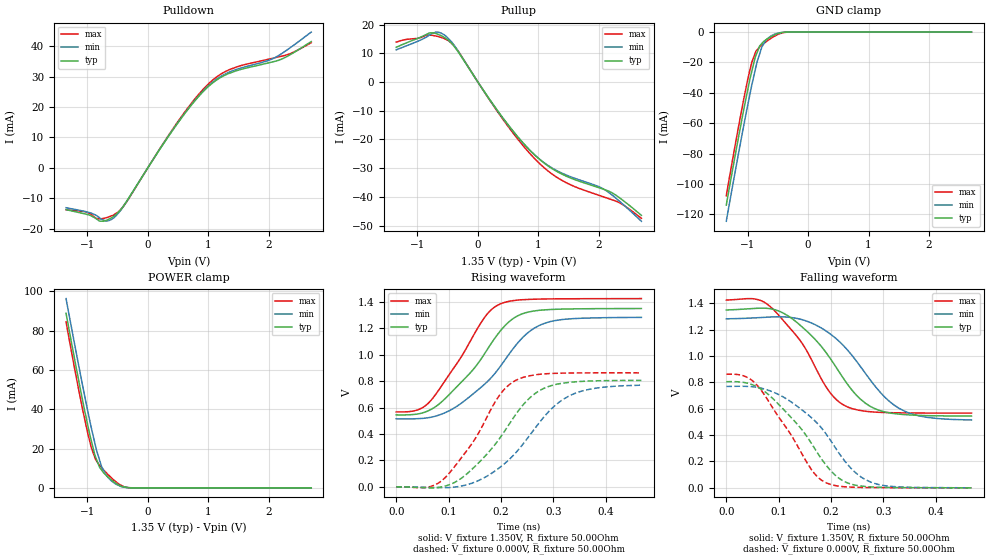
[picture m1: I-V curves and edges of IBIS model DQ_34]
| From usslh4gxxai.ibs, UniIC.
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| MODEL DQ_34 (34 Ohm Data I/O with no ODT, 800-2133Mbps)
[Model]   DQ_34
Model_type   I/O
Vinl = 545.000mV
Vinh = 805.000mV
Vmeas = 675.000mV
Vref = 675.000mV
Cref = 0.0pF
Rref = 25.000Ohm
|   typ   min   max
|C_comp   0.950pF   0.900pF   1.000pF
C_comp_pullup   0.4750pF   0.4500pF   0.5000pF
C_comp_pulldown   0.4750pF   0.4500pF   0.5000pF
[Model Spec]
| Input threshold voltage corners
Vinl   0.5450V   0.5115V   0.5825V
Vinh   0.8050V   0.7715V   0.8425V
| Measurement voltage corners
Vmeas   0.6750V   0.6415V   0.7125V
| Timing spec test load voltage corners
Vref   0.6750V   0.6415V   0.7125V
| Dynamic Overshoot Parameters from DDR3L Specification
|D_overshoot_ampl_h   0.40   NA   NA
|D_overshoot_ampl_l   0.40   NA   NA
|D_overshoot_area_h   0.11n   NA   NA
|D_overshoot_area_l   0.11n   NA   NA
[Receiver Thresholds]
Vth   =  0.675V
Vth_min  =  0.6615V
Vth_max  =  0.6885V
Vinh_ac  =  0.130V
Vinh_dc  =  0.090V
Vinl_ac  = -0.130V
Vinl_dc  = -0.090V
Tslew_ac =  5.000ns |Not specified, so set to high value
Threshold_sensitivity = 0.50
Reference_supply Pullup_ref
[Voltage Range]   1.3500V   1.2830V   1.4250V
[Pullup Reference]   1.3500V   1.2830V   1.4250V
[Temperature Range]   45.0   95.0   -40.0
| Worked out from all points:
|   slope of the pulldown table from 0 to 0.203 V, typ, clamps not added: 32.4 ohm
|   slope of the pullup table from 0 to 0.203 V, typ, clamps not added: 32.1 ohm
|   GND clamp passes 1 mA (typ) near -0.50 V on its own axis
|   POWER clamp passes 1 mA (typ) near -0.45 V on its own axis
|   falling waveform, V_fixture 1.350V, R_fixture 50.00Ohm: 20-80 % time 94.1ps typ, 97.5ps min, 82.7ps max; typ from 1.35 V to 0.545 V
|   rising waveform, V_fixture 1.350V, R_fixture 50.00Ohm: 20-80 % time 97.8ps typ, 105ps min, 81.4ps max; typ from 0.545 V to 1.35 V
|   rising waveform, V_fixture 0.000V, R_fixture 50.00Ohm: 20-80 % time 95.5ps typ, 103ps min, 81.4ps max; typ from 0 V to 0.806 V
|   falling waveform, V_fixture 0.000V, R_fixture 50.00Ohm: 20-80 % time 95.4ps typ, 100ps min, 81.6ps max; typ from 0.806 V to 0 V
[Pulldown]
|   Voltage   I(typ)   I(min)   I(max)
-1.35V    -13.75mA   -13.12mA   -13.81mA
-1V       -15.34mA   -14.53mA   -14.6mA
-800mV    -17.5mA    -16.38mA   -16.81mA
-690mV    -17.29mA   -17.5mA    -16.42mA
-565mV    -15.95mA   -16.5mA    -15.5mA
-395mV    -12.31mA   -12.44mA   -12.52mA
560mV     16.52mA    16.6mA     16.96mA
1.055V    27.67mA    27.92mA    28.56mA
1.465V    31.94mA    32.36mA    33.16mA
2.105V    35.05mA    36.27mA    36.22mA
2.34V     37.07mA    39.31mA    37.44mA
2.7V      41.52mA    44.64mA    41.15mA
[GND Clamp]
|   Voltage   I(typ)   I(min)   I(max)
-1.35V    -113.9mA   -124.5mA   -107.8mA
-1.205V   -81.48mA   -92.16mA   -74.7mA
-1.07V    -52.65mA   -63.14mA   -45.67mA
-1V       -38.7mA    -48.81mA   -31.8mA
-930mV    -25.95mA   -35.03mA   -20mA
-875mV    -16.88mA   -25.36mA   -14.11mA
-800mV    -9.222mA   -14.41mA   -9.781mA
-765mV    -7.604mA   -9.974mA   -8.618mA
-650mV    -3.918mA   -3.687mA   -5.173mA
-485mV    -837.4uA   -633.1uA   -1.288mA
-315mV    -19.67uA   -18.79uA   -29.52uA
2.7V      0A         0A         0A
[Pullup]
|   Voltage   I(typ)   I(min)   I(max)
-1.35V    12.15mA    11.27mA    13.95mA
-800mV    17.18mA    16.42mA    16.44mA
-690mV    16.9mA     17.47mA    16.07mA
-565mV    15.71mA    16.61mA    15.28mA
-320mV    10.4mA     10.59mA    10.63mA
470mV     -14.09mA   -14.2mA    -14.64mA
775mV     -21.88mA   -21.96mA   -22.88mA
1.055V    -27.57mA   -27.49mA   -29.11mA
1.465V    -32.85mA   -32.46mA   -35.14mA
2.105V    -37.57mA   -37.65mA   -40.24mA
2.34V     -40.35mA   -41.55mA   -42.07mA
2.7V      -46.46mA   -48.52mA   -47.48mA
[POWER Clamp]
|   Voltage   I(typ)   I(min)   I(max)
-1.35V    88.89mA    96.37mA    84.56mA
-1.205V   64.87mA    72.5mA     60.12mA
-1.07V    43.46mA    51mA       38.94mA
-930mV    23.58mA    30.09mA    20.17mA
-875mV    16.77mA    22.82mA    15.5mA
-800mV    10.68mA    14.43mA    11.57mA
-765mV    9.147mA    10.97mA    10.32mA
-690mV    6.433mA    6.617mA    7.805mA
-565mV    3.162mA    2.653mA    4.047mA
-395mV    485.8uA    358.5uA    553.6uA
-310mV    60.31uA    60.42uA    68.78uA
2.7V      0A         0A         0A
[Ramp]
R_load = 50.00Ohm
|   typ   min   max
dV/dt_r   483.363mV/95.498ps  461.741mV/103.129ps 517.629mV/81.416ps
dV/dt_f   483.183mV/94.118ps  460.840mV/97.492ps  514.663mV/82.746ps
[Falling Waveform]
V_fixture = 1.350V
V_fixture_min = 1.283V
V_fixture_max = 1.425V
R_fixture = 50.00Ohm
|   Time   V(typ)   V(min)   V(max)
0s        1.35V      1.283V     1.425V
54ps      1.362V     1.29V      1.434V
84ps      1.359V     1.296V     1.375V
162ps     1.157V     1.252V     977.6mV
198ps     984.4mV    1.169V     722.9mV
230ps     793.7mV    1.052V     616.4mV
274ps     620mV      823mV      577.8mV
328ps     560.3mV    607.7mV    569.4mV
382ps     548.1mV    535.9mV    567.6mV
468ps     544.7mV    514.9mV    567.2mV
[Rising Waveform]
V_fixture = 1.350V
V_fixture_min = 1.283V
V_fixture_max = 1.425V
R_fixture = 50.00Ohm
|   Time   V(typ)   V(min)   V(max)
0s        544.7mV    514.9mV    567.2mV
38ps      549.8mV    515.5mV    578.9mV
64ps      581mV      525.1mV    644.1mV
122ps     783.2mV    626.6mV    970.4mV
168ps     1.004V     774.3mV    1.279V
198ps     1.176V     907.7mV    1.383V
232ps     1.295V     1.089V     1.414V
280ps     1.339V     1.233V     1.422V
336ps     1.347V     1.273V     1.424V
468ps     1.35V      1.283V     1.425V
[Rising Waveform]
V_fixture = 0.000V
V_fixture_min = 0.000V
V_fixture_max = 0.000V
R_fixture = 50.00Ohm
|   Time   V(typ)   V(min)   V(max)
0s        -7.022uV   -2.894uV   8.588uV
58ps      -6.88mV    -4.479mV   -4.067mV
90ps      2.398mV    -6.977mV   57.05mV
158ps     184.2mV    49.04mV    412.4mV
198ps     369.9mV    147.2mV    697.5mV
230ps     558mV      266mV      809.5mV
274ps     729.5mV    490.1mV    852mV
328ps     789.6mV    683.7mV    861.4mV
382ps     802.6mV    747.6mV    862.9mV
468ps     805.6mV    769.6mV    862.7mV
[Falling Waveform]
V_fixture = 0.000V
V_fixture_min = 0.000V
V_fixture_max = 0.000V
R_fixture = 50.00Ohm
|   Time   V(typ)   V(min)   V(max)
0s        805.6mV    769.6mV    862.7mV
34ps      799.6mV    770.7mV    848.3mV
58ps      767.9mV    763.2mV    781.8mV
122ps     540.9mV    656.9mV    411.4mV
162ps     340mV      534.4mV    141.3mV
190ps     174.4mV    411.4mV    39.27mV
224ps     50.86mV    214.1mV    8.749mV
274ps     7.338mV    46.17mV    2.224mV
328ps     1.954mV    7.099mV    1.094mV
468ps     -7.022uV   -2.894uV   8.588uV
